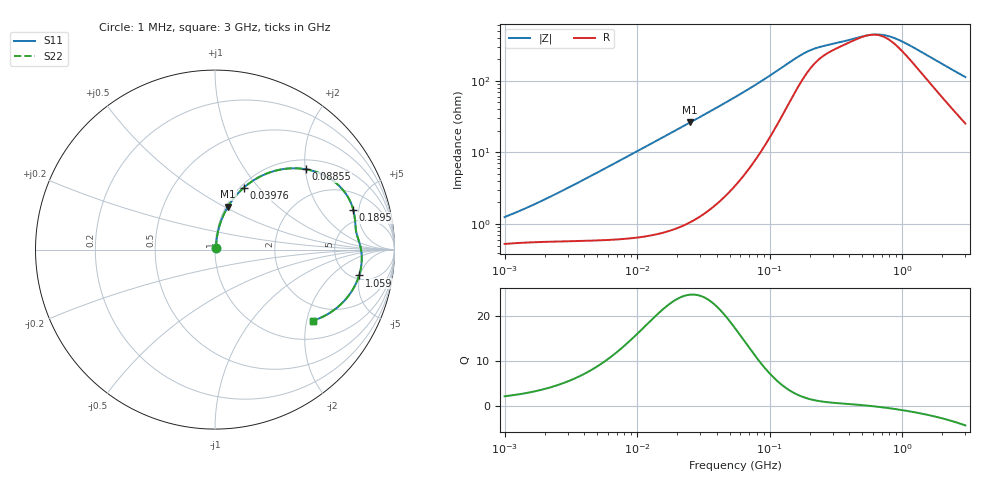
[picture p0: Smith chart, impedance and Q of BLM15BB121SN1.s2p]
! BLM15BB121SN1
# Hz S RI R 50
!Freq.(Hz) S11(Real) S11(Imag) S21(Real) S21(Imag) S12(Real) S12(Imag) S22(Real) S22(Imag)
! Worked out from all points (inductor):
!   401 points, 1 MHz to 3 GHz, reference 50 ohm
!   read as one part in series: L = 169 nH near 1.553 MHz
!   highest Q = 24.7 at 25.09 MHz (marker M1), where L = 166 nH
!   self-resonance near 577.4 MHz
!   S11 on the Smith chart (normalised r, x): 1 MHz: 1.01, +0.02; 39.76 MHz: 1.04, +0.84; 88.55 MHz: 1.22, +2.01; 189.5 MHz: 3.51, +4.35; 1.059 GHz: 5.62, -4.84; 3 GHz: 1.50, -2.19
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1000000  0.00537 0.0112  0.9946 -0.0112  0.9946 -0.0112  0.00537 0.0112
1751453  0.0059 0.0185  0.9941 -0.0185  0.9941 -0.0185  0.0059 0.0185
3823119  0.00733 0.0393  0.9927 -0.0393  0.9927 -0.0393  0.00733 0.0393
8017732  0.0129 0.0814  0.9871 -0.0814  0.9871 -0.0814  0.0129 0.0814
1.461624e7  0.0292 0.1459  0.9708 -0.1459  0.9708 -0.1459  0.0292 0.1459
2.509235e7  0.0725 0.2398  0.9275 -0.2398  0.9275 -0.2398  0.0725 0.2398
3.976269e7  0.1607 0.3454  0.8393 -0.3454  0.8393 -0.3454  0.1607 0.3454
5.477226e7  0.2694 0.4157  0.7306 -0.4157  0.7306 -0.4157  0.2694 0.4157
7.105049e7  0.3898 0.4499  0.6102 -0.4499  0.6102 -0.4499  0.3898 0.4499
8.854986e7  0.5058 0.4476  0.4942 -0.4476  0.4942 -0.4476  0.5058 0.4476
1.081723e8  0.6087 0.4141  0.3913 -0.4141  0.3913 -0.4141  0.6087 0.4141
1.321429e8  0.6932 0.3536  0.3068 -0.3536  0.3068 -0.3536  0.6932 0.3536
1.582265e8  0.7442 0.2868  0.2558 -0.2868  0.2558 -0.2868  0.7442 0.2868
1.894586e8  0.7704 0.2217  0.2296 -0.2217  0.2296 -0.2217  0.7704 0.2217
2.094008e8  0.7769 0.1902  0.2231 -0.1902  0.2231 -0.1902  0.7769 0.1902
2.716345e8  0.7824 0.1286  0.2176 -0.1286  0.2176 -0.1286  0.7824 0.1286
5.364635e8  0.8108 0.0146  0.1892 -0.0146  0.1892 -0.0146  0.8108 0.0146
6.553423e8  0.8169 -0.0268  0.1831 0.0268  0.1831 0.0268  0.8169 -0.0268
8.005644e8  0.8168 -0.0729  0.1832 0.0729  0.1832 0.0729  0.8168 -0.0729
1.059487e9  0.803 -0.1439  0.197 0.1439  0.197 0.1439  0.803 -0.1439
1.782824e9  0.7205 -0.2852  0.2795 0.2852  0.2795 0.2852  0.7205 -0.2852
3e9  0.5474 -0.3956  0.4526 0.3956  0.4526 0.3956  0.5474 -0.3956
